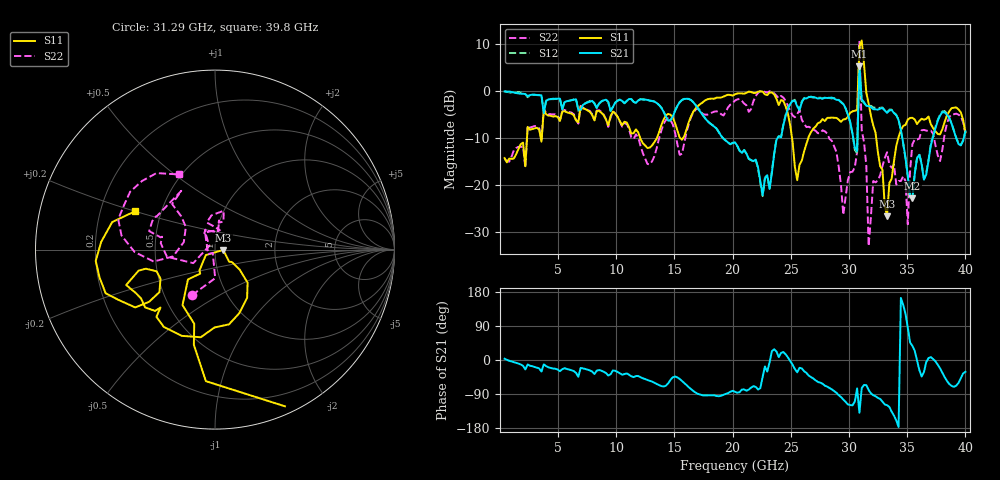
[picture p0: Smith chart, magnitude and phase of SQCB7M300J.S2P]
! Network Analyzer HP8722ES.07.66: Jul 25, 2000 Serial No. US39175408
! 27 Oct 2004  10:23:11
! Frequency  S11  S21  S12  S22
# HZ  S  DB R  50
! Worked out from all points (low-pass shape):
!   201 points, 400 MHz to 40 GHz, reference 50 ohm
!   highest |S21| = 5.24 dB at 30.89 GHz (marker M1); lowest = -22.9 dB at 35.45 GHz (marker M2)
!   |S21| within 3 dB of the highest: 30.85909 GHz to 30.97634 GHz (117.3 MHz wide, 0.379 % of centre)
!   lowest |S11| = -26.8 dB at 33.27 GHz (marker M3), VSWR 1.10, Z = 54.8 - j0.2 ohm
!   |S11| at or under -10 dB: start of sweep to 2.325 GHz; 12.05 GHz to 13.5 GHz (1.453 GHz wide, 11.4 % of centre); 32.33 GHz to 34.24 GHz (1.909 GHz wide, 5.73 % of centre)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
!   |S22| runs from -33.1 to 10.5 dB; largest |S21 - S12| = 0.098
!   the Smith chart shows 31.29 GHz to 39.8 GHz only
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4e8  -14.33 -90.0  -0.12 3.4  -0.04 4.6  -14.55 -85.6
7.132e9  -3.74 -106.8  -2.99 -22.1  -3.07 -23.0  -3.58 -113.8
1.3666e10  -8.89 -27.4  -3.00 -65.9  -2.95 -65.7  -10.19 -27.2
2.02e10  -0.73 -3.6  -10.98 -84.0  -11.01 -84.9  -2.06 -10.4
2.2576e10  -0.14 -22.7  -22.27 -44.4  -22.46 -42.2  0.03 -14.2
2.4358e10  -2.15 -64.9  -7.28 21.2  -7.05 20.5  -1.41 -38.6
2.5546e10  -19.05 54.4  -3.28 -32.4  -3.10 -33.4  -4.97 -28.2
2.6932e10  -8.03 93.8  -1.34 -48.9  -1.40 -51.6  -8.28 -34.8
2.8912e10  -5.76 59.5  -1.90 -86.4  -1.84 -88.5  -12.98 -52.5
2.9506e10  -6.08 56.6  -2.77 -104.4  -2.89 -105.5  -26.45 -11.3
3.0694e10  -4.07 43.5  -12.81 -75.0  -13.32 -74.3  -13.05 -136.5
3.0892e10  9.36 18.9  5.24 -139.2  4.80 -140.4  10.47 62.2
3.109e10  10.77 -45.2  -1.80 -74.2  -2.15 -73.0  -8.39 -161.3
3.1288e10  5.73 -69.6  -2.38 -65.9  -2.57 -63.4  -10.92 -116.8
3.1684e10  -2.68 -94.0  -3.25 -79.1  -3.14 -77.0  -33.12 -124.6
3.208e10  -7.35 -105.6  -3.90 -92.9  -3.50 -91.2  -19.23 120.5
3.3268e10  -26.78 -2.3  -4.66 -119.3  -4.57 -121.0  -13.08 77.4
3.3466e10  -19.62 -40.7  -4.16 -123.9  -3.98 -125.7  -15.74 73.1
3.505e10  -6.11 -99.2  -18.08 85.5  -18.26 83.8  -28.44 145.3
3.5446e10  -5.73 -123.5  -22.89 37.3  -22.76 33.1  -11.36 -171.5
3.802e10  -8.18 -142.6  -4.53 -33.5  -4.36 -35.2  -12.53 -170.8
4e10  -8.88 150.3  -8.61 -31.2  -8.54 -31.5  -9.00 104.1
